(* Logix 5000 AddOnInstructionDefinition export Banner_Q90R2_KD_Param_v4; software revision 33.00; part 2 of 3 *)
(* tags used below, declared in another part *)
   Q90R2KD : Banner_Q90R2KD_v4;
   Port_Data : Banner_IOL_Port_v4;
   Port : DINT;
   Local_Control : DINT;
   Command_Being_Processed : BOOL;
   Inprocess_Index : DINT;
(* Banner_Q90R2_KD_Param_v4, continued *)

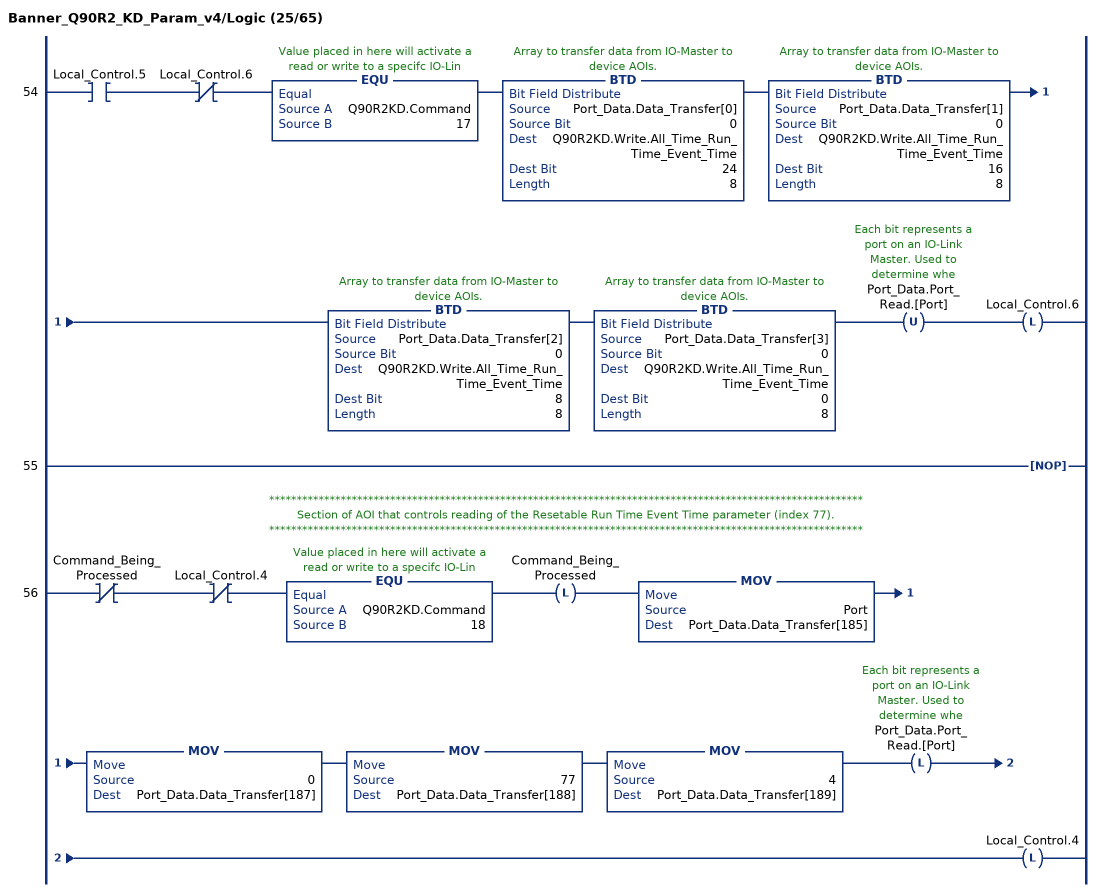
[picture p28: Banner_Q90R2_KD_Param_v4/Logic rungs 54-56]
   54: XIC(Local_Control.5)XIO(Local_Control.6)EQU(Q90R2KD.Command,17)BTD(Port_Data.Data_Transfer[0],0,Q90R2KD.Write.All_Time_Run_Time_Event_Time,24,8)BTD(Port_Data.Data_Transfer[1],0,Q90R2KD.Write.All_Time_Run_Time_Event_Time,16,8)BTD(Port_Data.Data_Transfer[2],0,Q90R2KD.Write.All_Time_Run_Time_Event_Time,8,8)BTD(Port_Data.Data_Transfer[3],0,Q90R2KD.Write.All_Time_Run_Time_Event_Time,0,8)OTU(Port_Data.Port_Read.[Port])OTL(Local_Control.6);
   55: NOP();
   // ************************************************************************************************************
   // Section of AOI that controls reading of the Resetable Run Time Event Time parameter (index 77).
   // ************************************************************************************************************
   56: XIO(Command_Being_Processed)XIO(Local_Control.4)EQU(Q90R2KD.Command,18)OTL(Command_Being_Processed)MOV(Port,Port_Data.Data_Transfer[185])MOV(0,Port_Data.Data_Transfer[187])MOV(77,Port_Data.Data_Transfer[188])MOV(4,Port_Data.Data_Transfer[189])OTL(Port_Data.Port_Read.[Port])OTL(Local_Control.4);
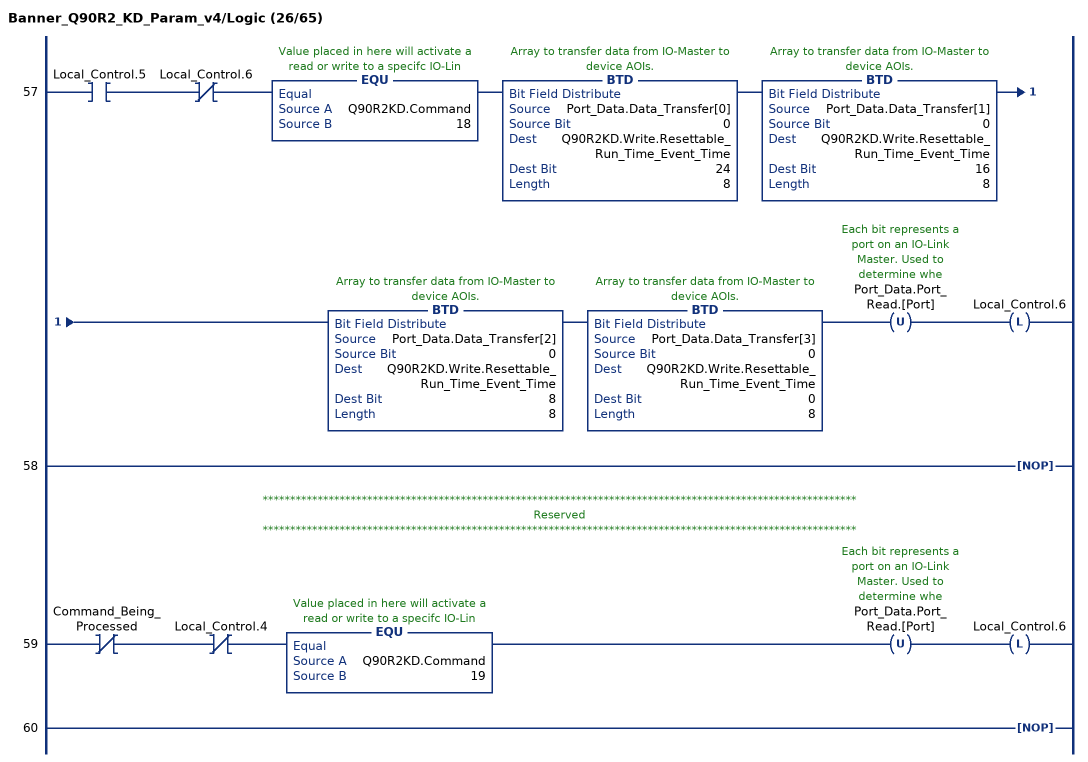
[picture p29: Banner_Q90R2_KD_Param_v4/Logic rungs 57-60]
   57: XIC(Local_Control.5)XIO(Local_Control.6)EQU(Q90R2KD.Command,18)BTD(Port_Data.Data_Transfer[0],0,Q90R2KD.Write.Resettable_Run_Time_Event_Time,24,8)BTD(Port_Data.Data_Transfer[1],0,Q90R2KD.Write.Resettable_Run_Time_Event_Time,16,8)BTD(Port_Data.Data_Transfer[2],0,Q90R2KD.Write.Resettable_Run_Time_Event_Time,8,8)BTD(Port_Data.Data_Transfer[3],0,Q90R2KD.Write.Resettable_Run_Time_Event_Time,0,8)OTU(Port_Data.Port_Read.[Port])OTL(Local_Control.6);
   58: NOP();
   // ************************************************************************************************************
   // Reserved
   // ************************************************************************************************************
   59: XIO(Command_Being_Processed)XIO(Local_Control.4)EQU(Q90R2KD.Command,19)OTU(Port_Data.Port_Read.[Port])OTL(Local_Control.6);
   60: NOP();
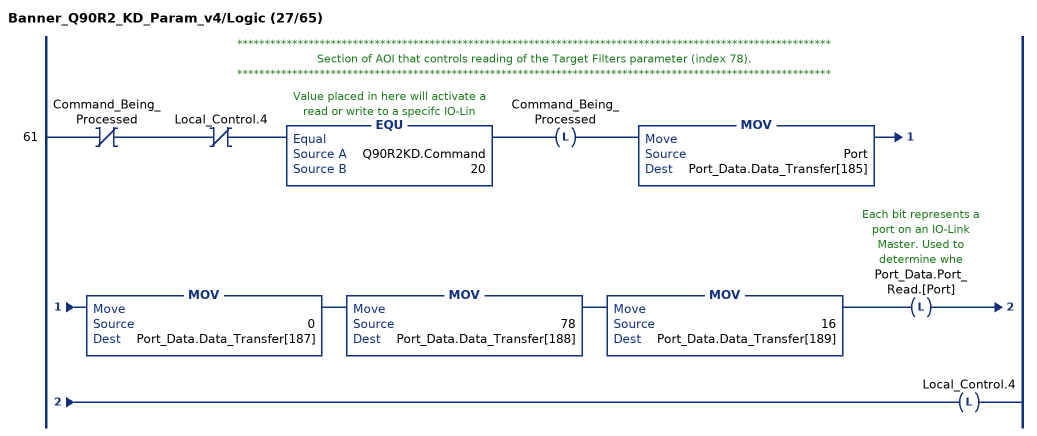
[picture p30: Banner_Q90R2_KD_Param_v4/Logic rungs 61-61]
   // ************************************************************************************************************
   // Section of AOI that controls reading of the Target Filters parameter (index 78).
   // ************************************************************************************************************
   61: XIO(Command_Being_Processed)XIO(Local_Control.4)EQU(Q90R2KD.Command,20)OTL(Command_Being_Processed)MOV(Port,Port_Data.Data_Transfer[185])MOV(0,Port_Data.Data_Transfer[187])MOV(78,Port_Data.Data_Transfer[188])MOV(16,Port_Data.Data_Transfer[189])OTL(Port_Data.Port_Read.[Port])OTL(Local_Control.4);
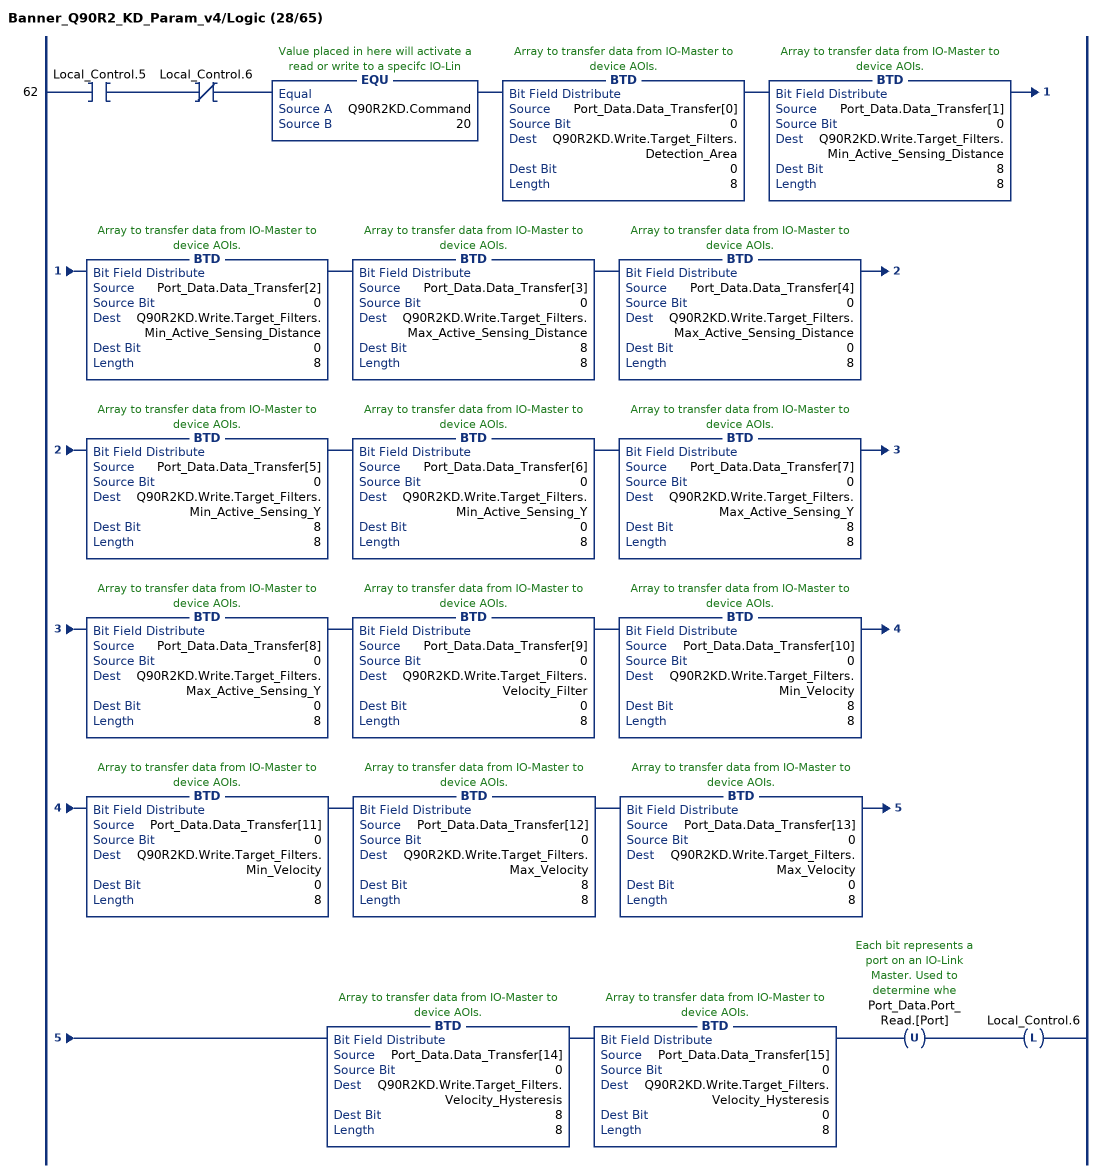
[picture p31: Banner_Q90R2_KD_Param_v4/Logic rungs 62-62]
   62: XIC(Local_Control.5)XIO(Local_Control.6)EQU(Q90R2KD.Command,20)BTD(Port_Data.Data_Transfer[0],0,Q90R2KD.Write.Target_Filters.Detection_Area,0,8)BTD(Port_Data.Data_Transfer[1],0,Q90R2KD.Write.Target_Filters.Min_Active_Sensing_Distance,8,8)BTD(Port_Data.Data_Transfer[2],0,Q90R2KD.Write.Target_Filters.Min_Active_Sensing_Distance,0,8)BTD(Port_Data.Data_Transfer[3],0,Q90R2KD.Write.Target_Filters.Max_Active_Sensing_Distance,8,8)BTD(Port_Data.Data_Transfer[4],0,Q90R2KD.Write.Target_Filters.Max_Active_Sensing_Distance,0,8)BTD(Port_Data.Data_Transfer[5],0,Q90R2KD.Write.Target_Filters.Min_Active_Sensing_Y,8,8)BTD(Port_Data.Data_Transfer[6],0,Q90R2KD.Write.Target_Filters.Min_Active_Sensing_Y,0,8)BTD(Port_Data.Data_Transfer[7],0,Q90R2KD.Write.Target_Filters.Max_Active_Sensing_Y,8,8)BTD(Port_Data.Data_Transfer[8],0,Q90R2KD.Write.Target_Filters.Max_Active_Sensing_Y,0,8)BTD(Port_Data.Data_Transfer[9],0,Q90R2KD.Write.Target_Filters.Velocity_Filter,0,8)BTD(Port_Data.Data_Transfer[10],0,Q90R2KD.Write.Target_Filters.Min_Velocity,8,8)BTD(Port_Data.Data_Transfer[11],0,Q90R2KD.Write.Target_Filters.Min_Velocity,0,8)BTD(Port_Data.Data_Transfer[12],0,Q90R2KD.Write.Target_Filters.Max_Velocity,8,8)BTD(Port_Data.Data_Transfer[13],0,Q90R2KD.Write.Target_Filters.Max_Velocity,0,8)BTD(Port_Data.Data_Transfer[14],0,Q90R2KD.Write.Target_Filters.Velocity_Hysteresis,8,8)BTD(Port_Data.Data_Transfer[15],0,Q90R2KD.Write.Target_Filters.Velocity_Hysteresis,0,8)OTU(Port_Data.Port_Read.[Port])OTL(Local_Control.6);
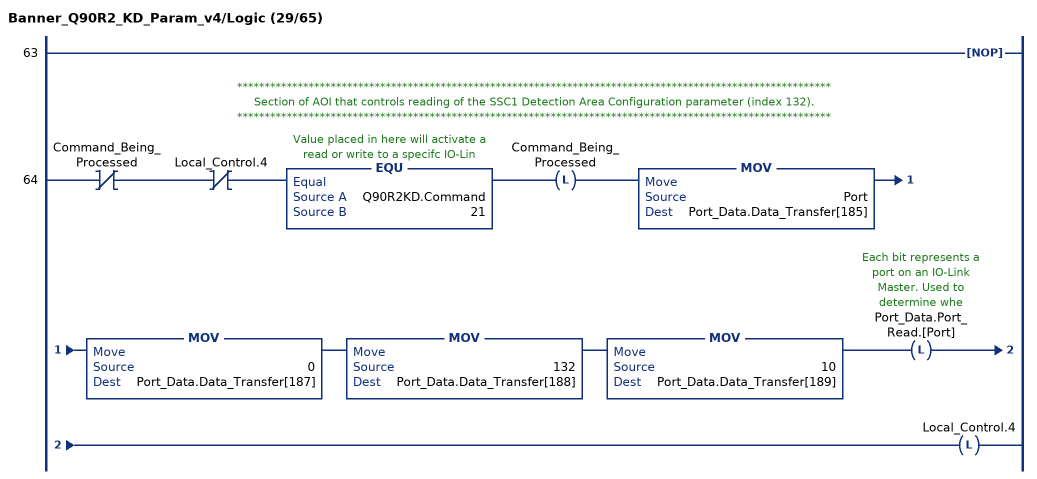
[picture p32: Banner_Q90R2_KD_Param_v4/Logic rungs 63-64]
   63: NOP();
   // ************************************************************************************************************
   // Section of AOI that controls reading of the SSC1 Detection Area Configuration parameter (index 132).
   // ************************************************************************************************************
   64: XIO(Command_Being_Processed)XIO(Local_Control.4)EQU(Q90R2KD.Command,21)OTL(Command_Being_Processed)MOV(Port,Port_Data.Data_Transfer[185])MOV(0,Port_Data.Data_Transfer[187])MOV(132,Port_Data.Data_Transfer[188])MOV(10,Port_Data.Data_Transfer[189])OTL(Port_Data.Port_Read.[Port])OTL(Local_Control.4);
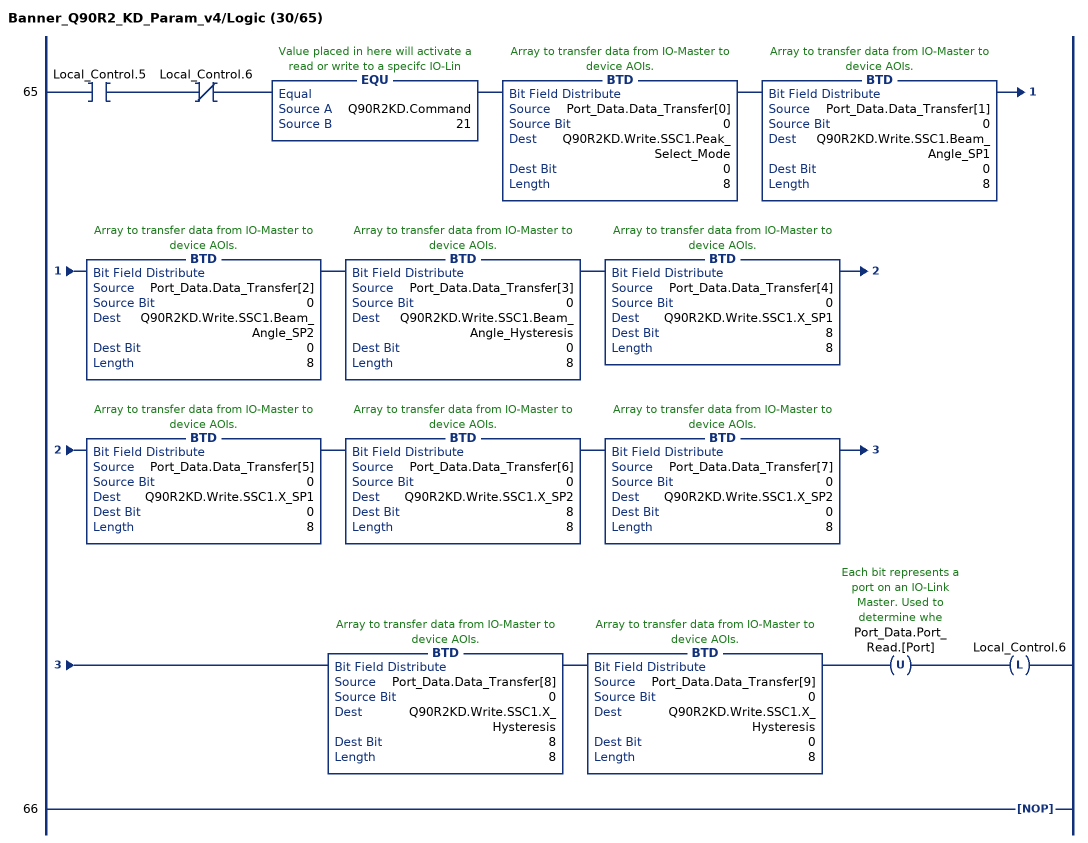
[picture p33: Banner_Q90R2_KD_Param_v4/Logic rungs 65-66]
   65: XIC(Local_Control.5)XIO(Local_Control.6)EQU(Q90R2KD.Command,21)BTD(Port_Data.Data_Transfer[0],0,Q90R2KD.Write.SSC1.Peak_Select_Mode,0,8)BTD(Port_Data.Data_Transfer[1],0,Q90R2KD.Write.SSC1.Beam_Angle_SP1,0,8)BTD(Port_Data.Data_Transfer[2],0,Q90R2KD.Write.SSC1.Beam_Angle_SP2,0,8)BTD(Port_Data.Data_Transfer[3],0,Q90R2KD.Write.SSC1.Beam_Angle_Hysteresis,0,8)BTD(Port_Data.Data_Transfer[4],0,Q90R2KD.Write.SSC1.X_SP1,8,8)BTD(Port_Data.Data_Transfer[5],0,Q90R2KD.Write.SSC1.X_SP1,0,8)BTD(Port_Data.Data_Transfer[6],0,Q90R2KD.Write.SSC1.X_SP2,8,8)BTD(Port_Data.Data_Transfer[7],0,Q90R2KD.Write.SSC1.X_SP2,0,8)BTD(Port_Data.Data_Transfer[8],0,Q90R2KD.Write.SSC1.X_Hysteresis,8,8)BTD(Port_Data.Data_Transfer[9],0,Q90R2KD.Write.SSC1.X_Hysteresis,0,8)OTU(Port_Data.Port_Read.[Port])OTL(Local_Control.6);
   66: NOP();
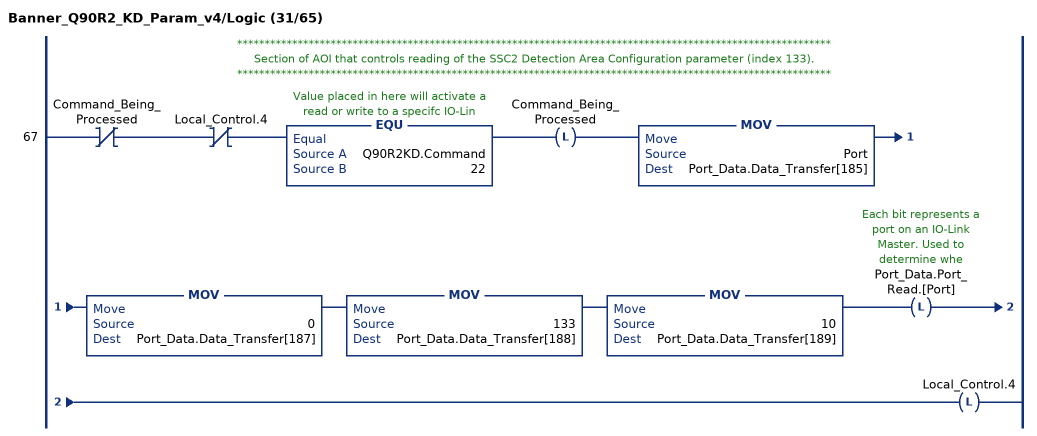
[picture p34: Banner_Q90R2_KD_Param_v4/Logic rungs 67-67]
   // ************************************************************************************************************
   // Section of AOI that controls reading of the SSC2 Detection Area Configuration parameter (index 133).
   // ************************************************************************************************************
   67: XIO(Command_Being_Processed)XIO(Local_Control.4)EQU(Q90R2KD.Command,22)OTL(Command_Being_Processed)MOV(Port,Port_Data.Data_Transfer[185])MOV(0,Port_Data.Data_Transfer[187])MOV(133,Port_Data.Data_Transfer[188])MOV(10,Port_Data.Data_Transfer[189])OTL(Port_Data.Port_Read.[Port])OTL(Local_Control.4);
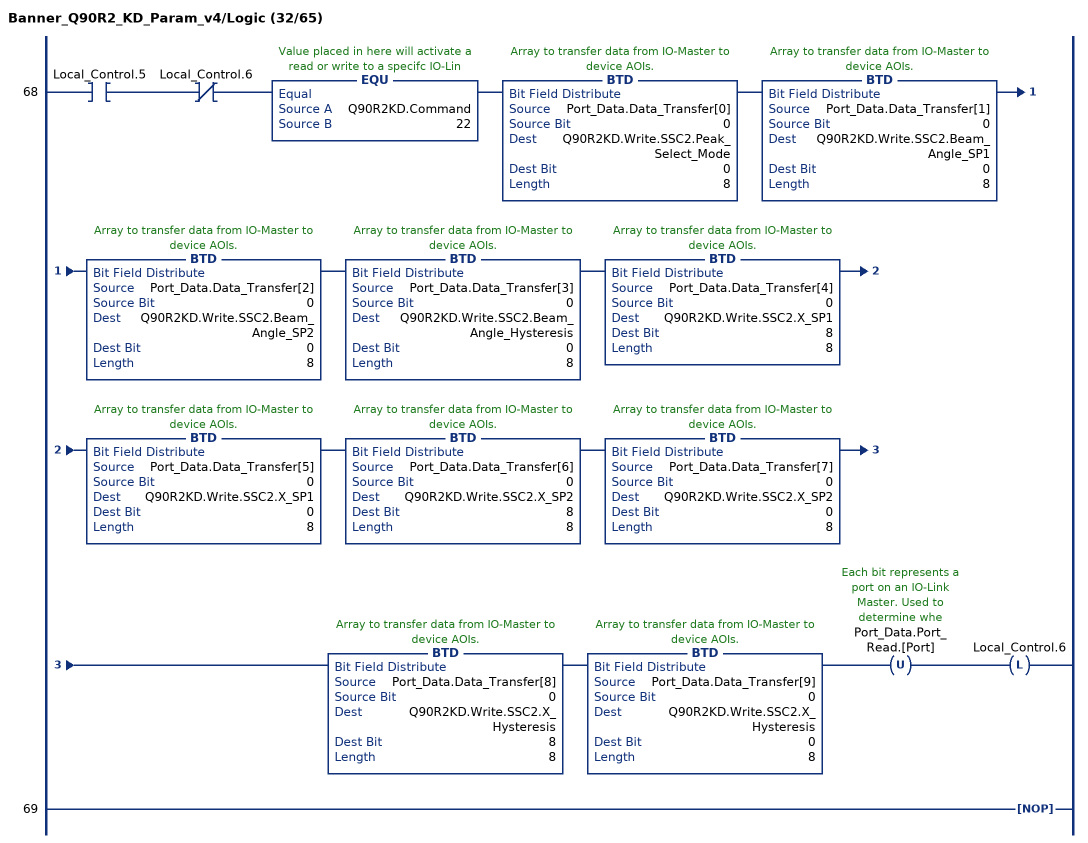
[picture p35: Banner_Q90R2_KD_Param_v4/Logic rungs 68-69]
   68: XIC(Local_Control.5)XIO(Local_Control.6)EQU(Q90R2KD.Command,22)BTD(Port_Data.Data_Transfer[0],0,Q90R2KD.Write.SSC2.Peak_Select_Mode,0,8)BTD(Port_Data.Data_Transfer[1],0,Q90R2KD.Write.SSC2.Beam_Angle_SP1,0,8)BTD(Port_Data.Data_Transfer[2],0,Q90R2KD.Write.SSC2.Beam_Angle_SP2,0,8)BTD(Port_Data.Data_Transfer[3],0,Q90R2KD.Write.SSC2.Beam_Angle_Hysteresis,0,8)BTD(Port_Data.Data_Transfer[4],0,Q90R2KD.Write.SSC2.X_SP1,8,8)BTD(Port_Data.Data_Transfer[5],0,Q90R2KD.Write.SSC2.X_SP1,0,8)BTD(Port_Data.Data_Transfer[6],0,Q90R2KD.Write.SSC2.X_SP2,8,8)BTD(Port_Data.Data_Transfer[7],0,Q90R2KD.Write.SSC2.X_SP2,0,8)BTD(Port_Data.Data_Transfer[8],0,Q90R2KD.Write.SSC2.X_Hysteresis,8,8)BTD(Port_Data.Data_Transfer[9],0,Q90R2KD.Write.SSC2.X_Hysteresis,0,8)OTU(Port_Data.Port_Read.[Port])OTL(Local_Control.6);
   69: NOP();
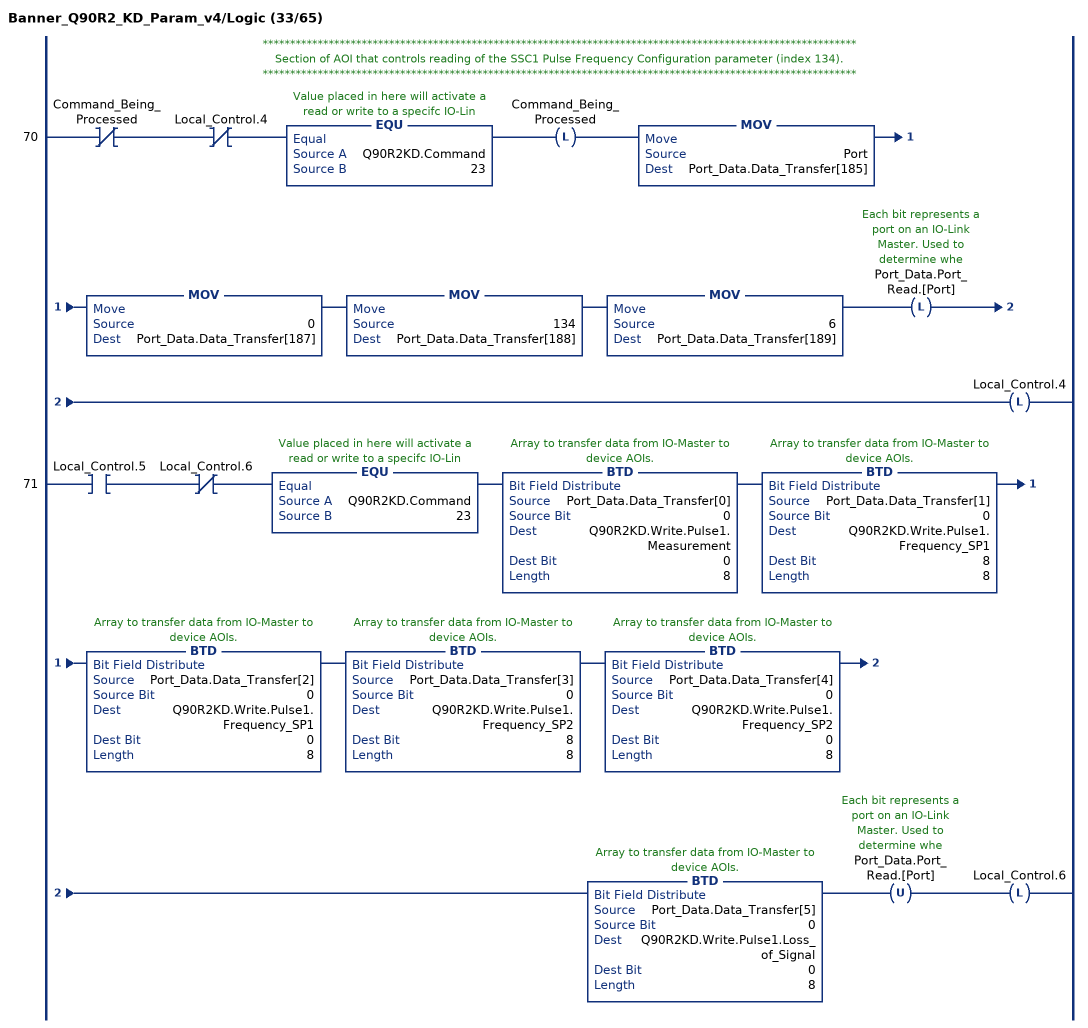
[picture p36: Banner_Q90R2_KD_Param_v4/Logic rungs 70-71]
   // ************************************************************************************************************
   // Section of AOI that controls reading of the SSC1 Pulse Frequency Configuration parameter (index 134).
   // ************************************************************************************************************
   70: XIO(Command_Being_Processed)XIO(Local_Control.4)EQU(Q90R2KD.Command,23)OTL(Command_Being_Processed)MOV(Port,Port_Data.Data_Transfer[185])MOV(0,Port_Data.Data_Transfer[187])MOV(134,Port_Data.Data_Transfer[188])MOV(6,Port_Data.Data_Transfer[189])OTL(Port_Data.Port_Read.[Port])OTL(Local_Control.4);
   71: XIC(Local_Control.5)XIO(Local_Control.6)EQU(Q90R2KD.Command,23)BTD(Port_Data.Data_Transfer[0],0,Q90R2KD.Write.Pulse1.Measurement,0,8)BTD(Port_Data.Data_Transfer[1],0,Q90R2KD.Write.Pulse1.Frequency_SP1,8,8)BTD(Port_Data.Data_Transfer[2],0,Q90R2KD.Write.Pulse1.Frequency_SP1,0,8)BTD(Port_Data.Data_Transfer[3],0,Q90R2KD.Write.Pulse1.Frequency_SP2,8,8)BTD(Port_Data.Data_Transfer[4],0,Q90R2KD.Write.Pulse1.Frequency_SP2,0,8)BTD(Port_Data.Data_Transfer[5],0,Q90R2KD.Write.Pulse1.Loss_of_Signal,0,8)OTU(Port_Data.Port_Read.[Port])OTL(Local_Control.6);
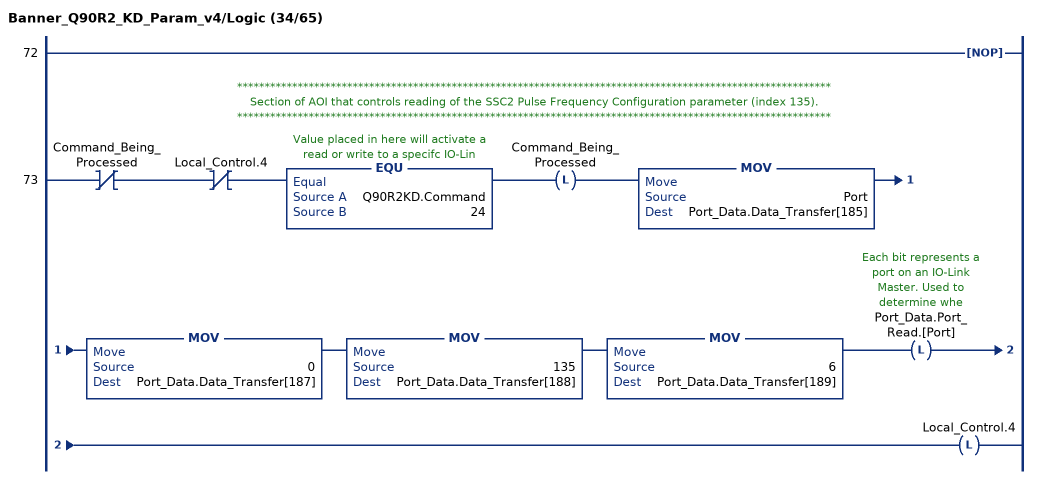
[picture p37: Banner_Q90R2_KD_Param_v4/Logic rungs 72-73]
   72: NOP();
   // ************************************************************************************************************
   // Section of AOI that controls reading of the SSC2 Pulse Frequency Configuration parameter (index 135).
   // ************************************************************************************************************
   73: XIO(Command_Being_Processed)XIO(Local_Control.4)EQU(Q90R2KD.Command,24)OTL(Command_Being_Processed)MOV(Port,Port_Data.Data_Transfer[185])MOV(0,Port_Data.Data_Transfer[187])MOV(135,Port_Data.Data_Transfer[188])MOV(6,Port_Data.Data_Transfer[189])OTL(Port_Data.Port_Read.[Port])OTL(Local_Control.4);
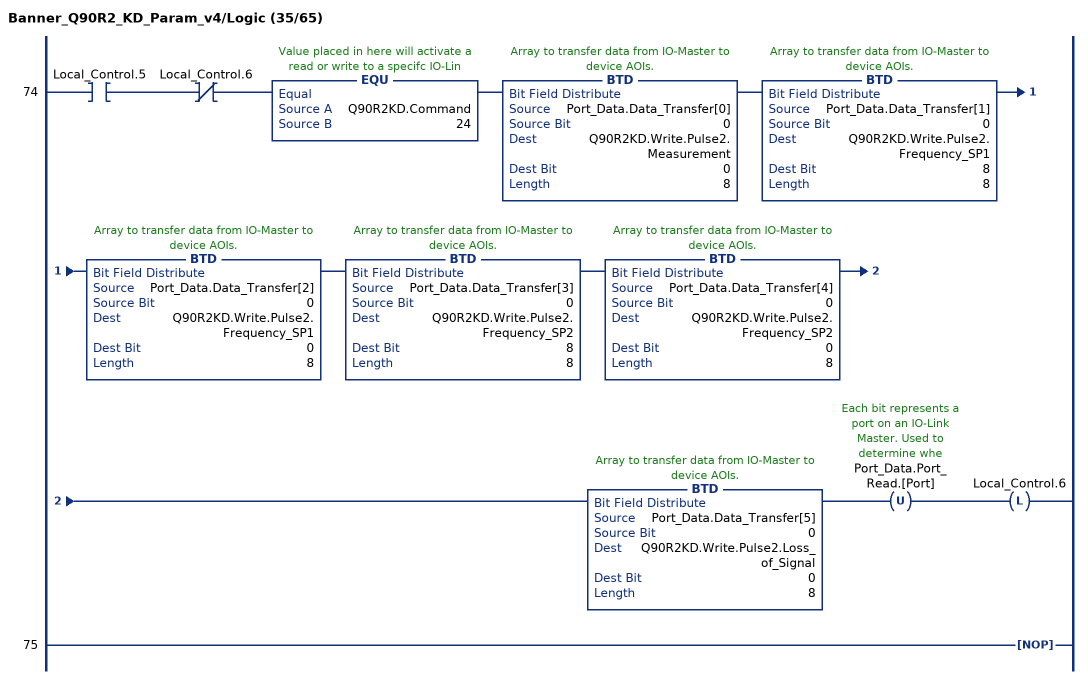
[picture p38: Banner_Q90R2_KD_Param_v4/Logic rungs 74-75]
   74: XIC(Local_Control.5)XIO(Local_Control.6)EQU(Q90R2KD.Command,24)BTD(Port_Data.Data_Transfer[0],0,Q90R2KD.Write.Pulse2.Measurement,0,8)BTD(Port_Data.Data_Transfer[1],0,Q90R2KD.Write.Pulse2.Frequency_SP1,8,8)BTD(Port_Data.Data_Transfer[2],0,Q90R2KD.Write.Pulse2.Frequency_SP1,0,8)BTD(Port_Data.Data_Transfer[3],0,Q90R2KD.Write.Pulse2.Frequency_SP2,8,8)BTD(Port_Data.Data_Transfer[4],0,Q90R2KD.Write.Pulse2.Frequency_SP2,0,8)BTD(Port_Data.Data_Transfer[5],0,Q90R2KD.Write.Pulse2.Loss_of_Signal,0,8)OTU(Port_Data.Port_Read.[Port])OTL(Local_Control.6);
   75: NOP();
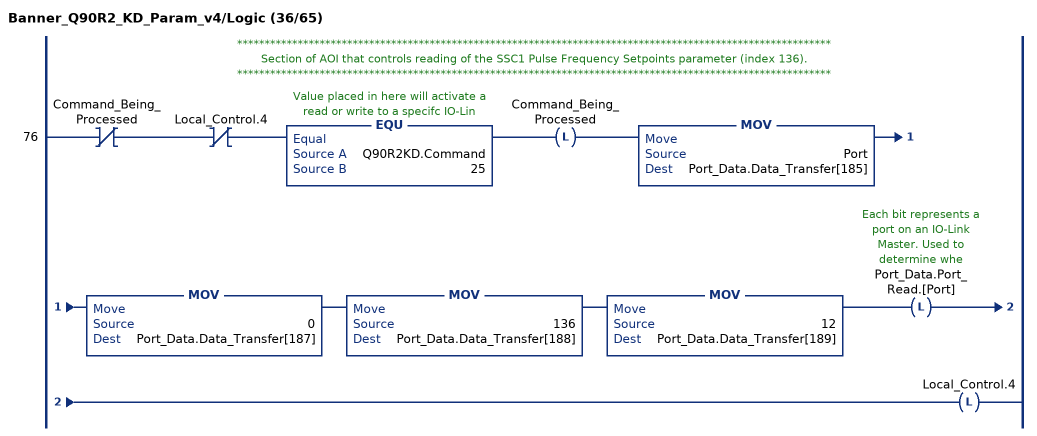
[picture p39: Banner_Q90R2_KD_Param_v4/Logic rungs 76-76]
   // ************************************************************************************************************
   // Section of AOI that controls reading of the SSC1 Pulse Frequency Setpoints parameter (index 136).
   // ************************************************************************************************************
   76: XIO(Command_Being_Processed)XIO(Local_Control.4)EQU(Q90R2KD.Command,25)OTL(Command_Being_Processed)MOV(Port,Port_Data.Data_Transfer[185])MOV(0,Port_Data.Data_Transfer[187])MOV(136,Port_Data.Data_Transfer[188])MOV(12,Port_Data.Data_Transfer[189])OTL(Port_Data.Port_Read.[Port])OTL(Local_Control.4);
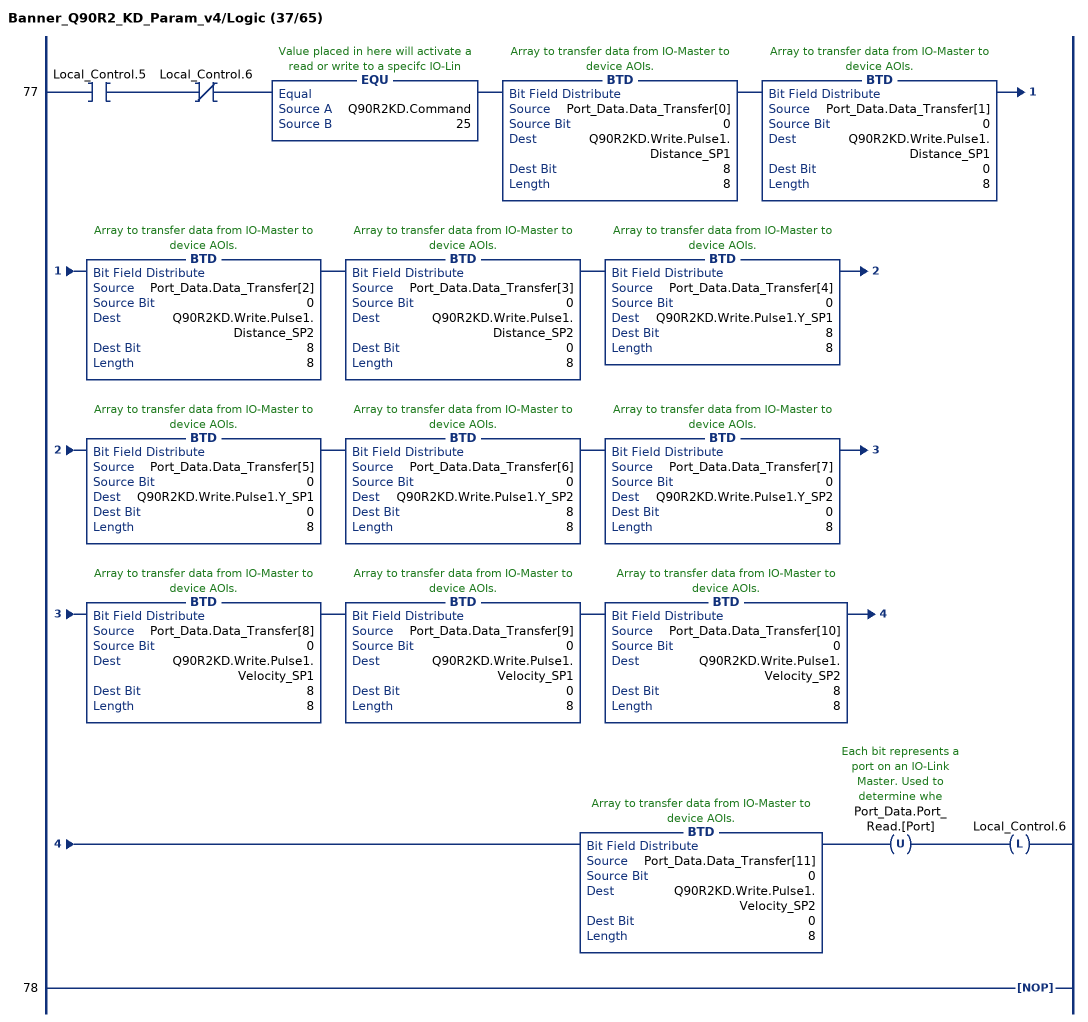
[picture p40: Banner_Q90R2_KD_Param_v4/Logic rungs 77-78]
   77: XIC(Local_Control.5)XIO(Local_Control.6)EQU(Q90R2KD.Command,25)BTD(Port_Data.Data_Transfer[0],0,Q90R2KD.Write.Pulse1.Distance_SP1,8,8)BTD(Port_Data.Data_Transfer[1],0,Q90R2KD.Write.Pulse1.Distance_SP1,0,8)BTD(Port_Data.Data_Transfer[2],0,Q90R2KD.Write.Pulse1.Distance_SP2,8,8)BTD(Port_Data.Data_Transfer[3],0,Q90R2KD.Write.Pulse1.Distance_SP2,0,8)BTD(Port_Data.Data_Transfer[4],0,Q90R2KD.Write.Pulse1.Y_SP1,8,8)BTD(Port_Data.Data_Transfer[5],0,Q90R2KD.Write.Pulse1.Y_SP1,0,8)BTD(Port_Data.Data_Transfer[6],0,Q90R2KD.Write.Pulse1.Y_SP2,8,8)BTD(Port_Data.Data_Transfer[7],0,Q90R2KD.Write.Pulse1.Y_SP2,0,8)BTD(Port_Data.Data_Transfer[8],0,Q90R2KD.Write.Pulse1.Velocity_SP1,8,8)BTD(Port_Data.Data_Transfer[9],0,Q90R2KD.Write.Pulse1.Velocity_SP1,0,8)BTD(Port_Data.Data_Transfer[10],0,Q90R2KD.Write.Pulse1.Velocity_SP2,8,8)BTD(Port_Data.Data_Transfer[11],0,Q90R2KD.Write.Pulse1.Velocity_SP2,0,8)OTU(Port_Data.Port_Read.[Port])OTL(Local_Control.6);
   78: NOP();
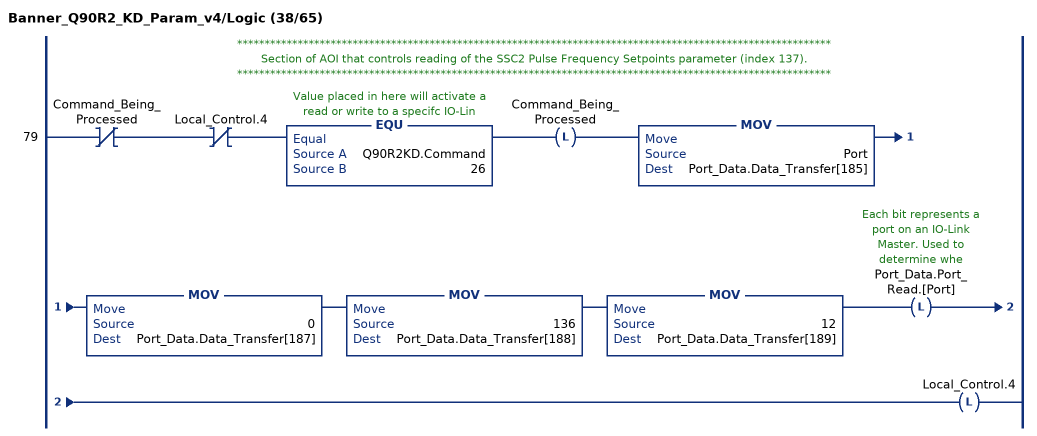
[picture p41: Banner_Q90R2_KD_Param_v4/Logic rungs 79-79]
   // ************************************************************************************************************
   // Section of AOI that controls reading of the SSC2 Pulse Frequency Setpoints parameter (index 137).
   // ************************************************************************************************************
   79: XIO(Command_Being_Processed)XIO(Local_Control.4)EQU(Q90R2KD.Command,26)OTL(Command_Being_Processed)MOV(Port,Port_Data.Data_Transfer[185])MOV(0,Port_Data.Data_Transfer[187])MOV(136,Port_Data.Data_Transfer[188])MOV(12,Port_Data.Data_Transfer[189])OTL(Port_Data.Port_Read.[Port])OTL(Local_Control.4);
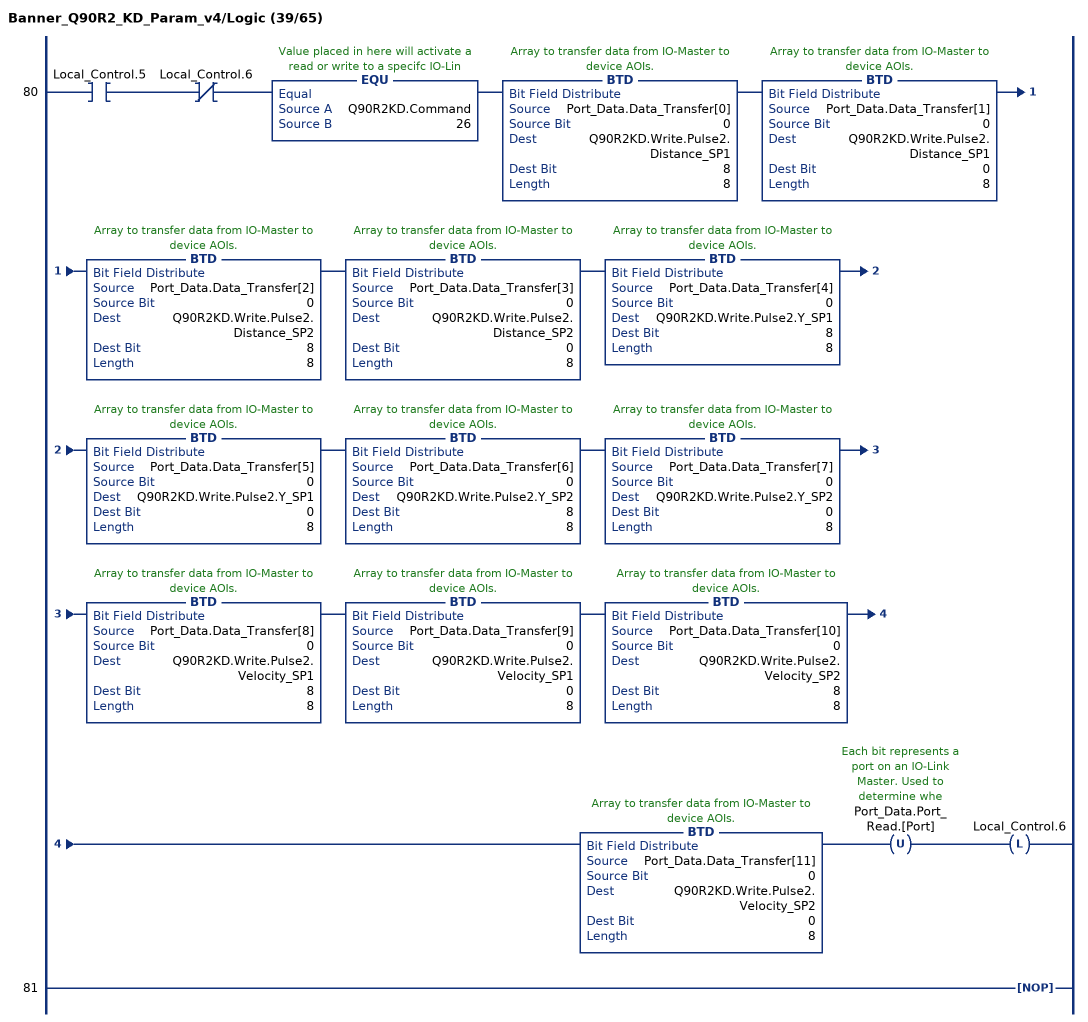
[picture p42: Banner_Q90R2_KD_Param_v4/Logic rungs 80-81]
   80: XIC(Local_Control.5)XIO(Local_Control.6)EQU(Q90R2KD.Command,26)BTD(Port_Data.Data_Transfer[0],0,Q90R2KD.Write.Pulse2.Distance_SP1,8,8)BTD(Port_Data.Data_Transfer[1],0,Q90R2KD.Write.Pulse2.Distance_SP1,0,8)BTD(Port_Data.Data_Transfer[2],0,Q90R2KD.Write.Pulse2.Distance_SP2,8,8)BTD(Port_Data.Data_Transfer[3],0,Q90R2KD.Write.Pulse2.Distance_SP2,0,8)BTD(Port_Data.Data_Transfer[4],0,Q90R2KD.Write.Pulse2.Y_SP1,8,8)BTD(Port_Data.Data_Transfer[5],0,Q90R2KD.Write.Pulse2.Y_SP1,0,8)BTD(Port_Data.Data_Transfer[6],0,Q90R2KD.Write.Pulse2.Y_SP2,8,8)BTD(Port_Data.Data_Transfer[7],0,Q90R2KD.Write.Pulse2.Y_SP2,0,8)BTD(Port_Data.Data_Transfer[8],0,Q90R2KD.Write.Pulse2.Velocity_SP1,8,8)BTD(Port_Data.Data_Transfer[9],0,Q90R2KD.Write.Pulse2.Velocity_SP1,0,8)BTD(Port_Data.Data_Transfer[10],0,Q90R2KD.Write.Pulse2.Velocity_SP2,8,8)BTD(Port_Data.Data_Transfer[11],0,Q90R2KD.Write.Pulse2.Velocity_SP2,0,8)OTU(Port_Data.Port_Read.[Port])OTL(Local_Control.6);
   81: NOP();
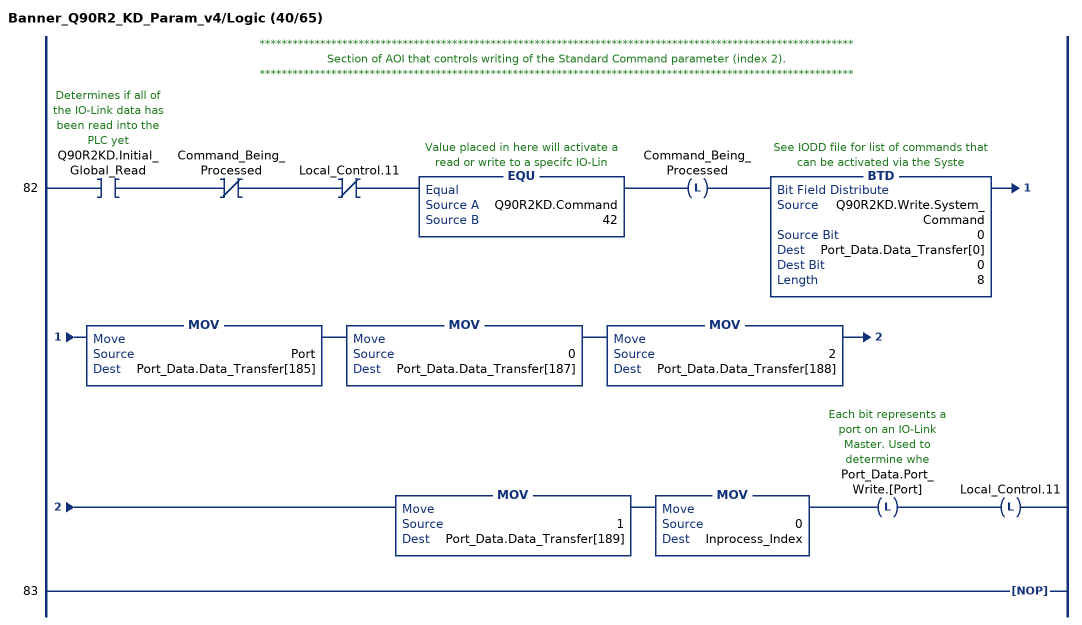
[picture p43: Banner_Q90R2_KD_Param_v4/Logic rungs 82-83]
   // ************************************************************************************************************
   // Section of AOI that controls writing of the Standard Command parameter (index 2).
   // ************************************************************************************************************
   82: XIC(Q90R2KD.Initial_Global_Read)XIO(Command_Being_Processed)XIO(Local_Control.11)EQU(Q90R2KD.Command,42)OTL(Command_Being_Processed)BTD(Q90R2KD.Write.System_Command,0,Port_Data.Data_Transfer[0],0,8)MOV(Port,Port_Data.Data_Transfer[185])MOV(0,Port_Data.Data_Transfer[187])MOV(2,Port_Data.Data_Transfer[188])MOV(1,Port_Data.Data_Transfer[189])MOV(0,Inprocess_Index)OTL(Port_Data.Port_Write.[Port])OTL(Local_Control.11);
   83: NOP();
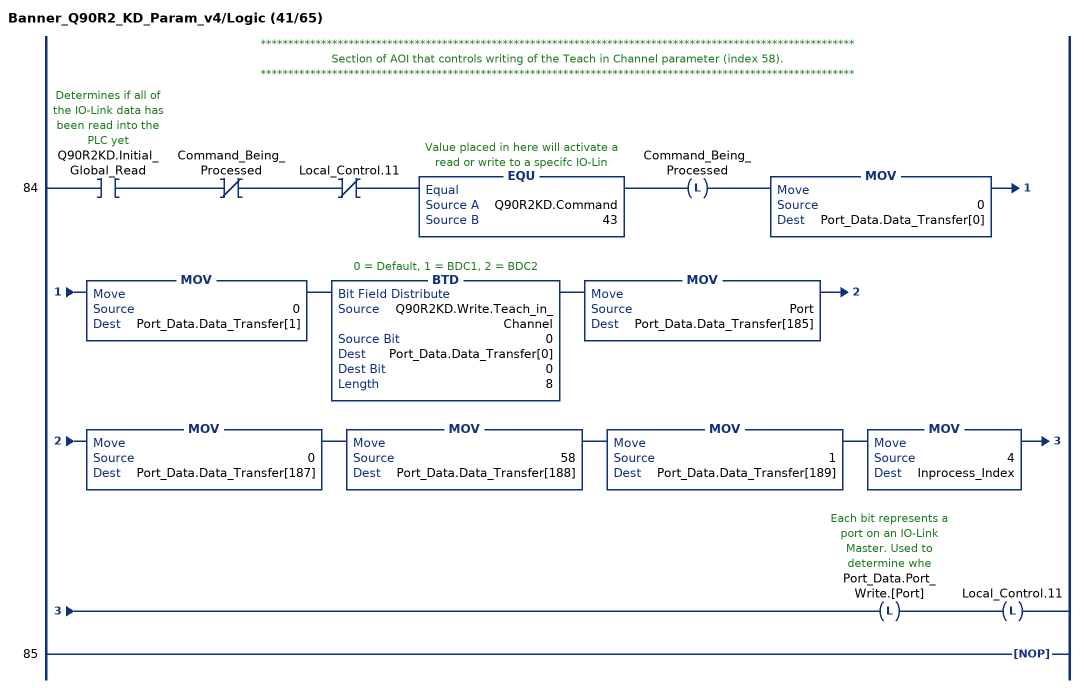
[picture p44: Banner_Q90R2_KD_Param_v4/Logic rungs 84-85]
   // ************************************************************************************************************
   // Section of AOI that controls writing of the Teach in Channel parameter (index 58).
   // ************************************************************************************************************
   84: XIC(Q90R2KD.Initial_Global_Read)XIO(Command_Being_Processed)XIO(Local_Control.11)EQU(Q90R2KD.Command,43)OTL(Command_Being_Processed)MOV(0,Port_Data.Data_Transfer[0])MOV(0,Port_Data.Data_Transfer[1])BTD(Q90R2KD.Write.Teach_in_Channel,0,Port_Data.Data_Transfer[0],0,8)MOV(Port,Port_Data.Data_Transfer[185])MOV(0,Port_Data.Data_Transfer[187])MOV(58,Port_Data.Data_Transfer[188])MOV(1,Port_Data.Data_Transfer[189])MOV(4,Inprocess_Index)OTL(Port_Data.Port_Write.[Port])OTL(Local_Control.11);
   85: NOP();
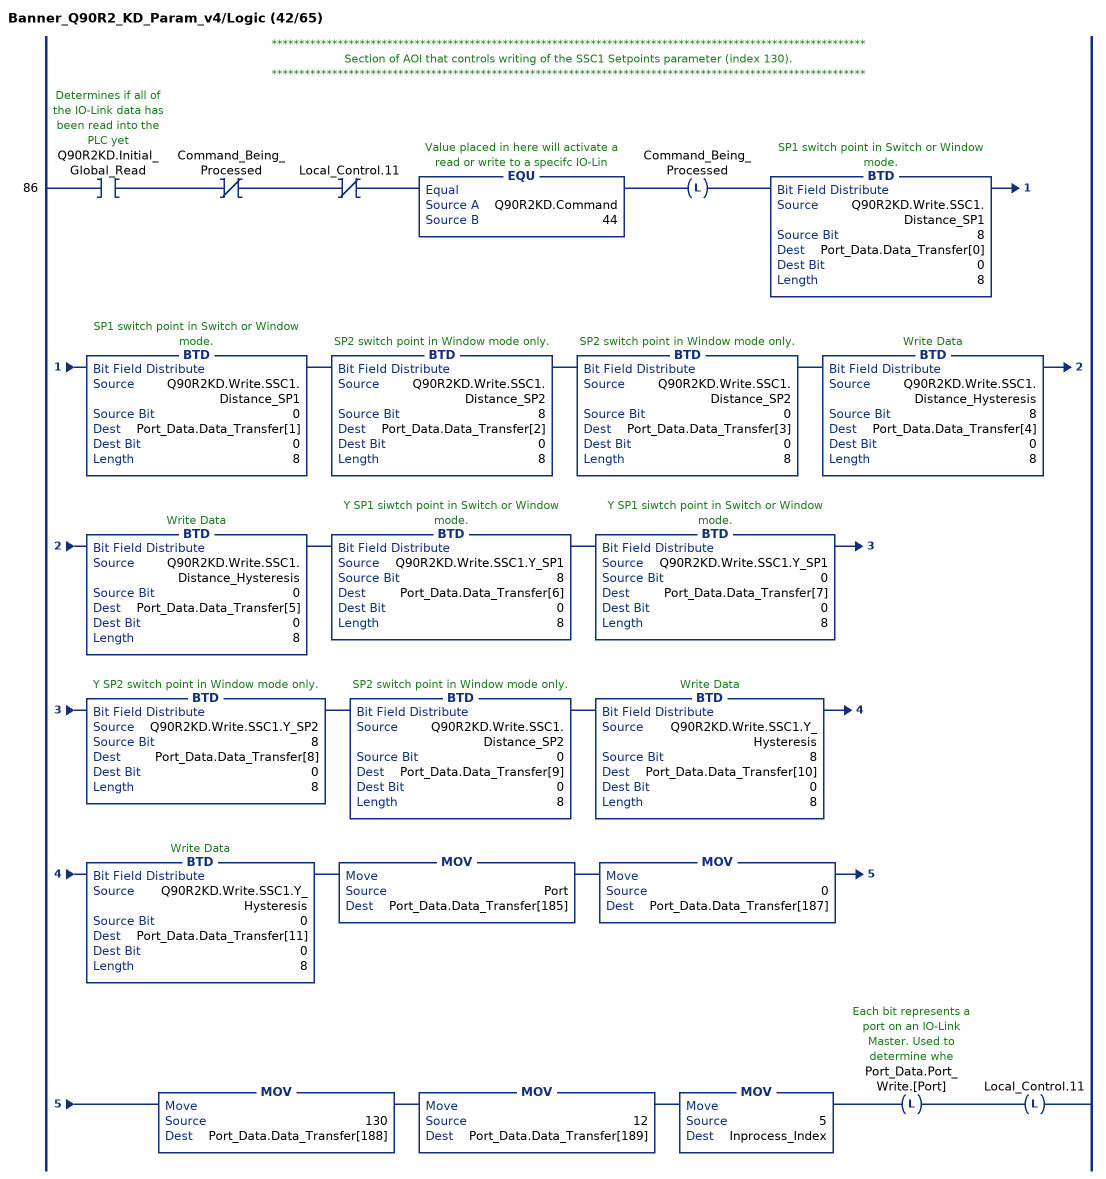
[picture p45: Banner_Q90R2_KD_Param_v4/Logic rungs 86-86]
   // ************************************************************************************************************
   // Section of AOI that controls writing of the SSC1 Setpoints parameter (index 130).
   // ************************************************************************************************************
   86: XIC(Q90R2KD.Initial_Global_Read)XIO(Command_Being_Processed)XIO(Local_Control.11)EQU(Q90R2KD.Command,44)OTL(Command_Being_Processed)BTD(Q90R2KD.Write.SSC1.Distance_SP1,8,Port_Data.Data_Transfer[0],0,8)BTD(Q90R2KD.Write.SSC1.Distance_SP1,0,Port_Data.Data_Transfer[1],0,8)BTD(Q90R2KD.Write.SSC1.Distance_SP2,8,Port_Data.Data_Transfer[2],0,8)BTD(Q90R2KD.Write.SSC1.Distance_SP2,0,Port_Data.Data_Transfer[3],0,8)BTD(Q90R2KD.Write.SSC1.Distance_Hysteresis,8,Port_Data.Data_Transfer[4],0,8)BTD(Q90R2KD.Write.SSC1.Distance_Hysteresis,0,Port_Data.Data_Transfer[5],0,8)BTD(Q90R2KD.Write.SSC1.Y_SP1,8,Port_Data.Data_Transfer[6],0,8)BTD(Q90R2KD.Write.SSC1.Y_SP1,0,Port_Data.Data_Transfer[7],0,8)BTD(Q90R2KD.Write.SSC1.Y_SP2,8,Port_Data.Data_Transfer[8],0,8)BTD(Q90R2KD.Write.SSC1.Distance_SP2,0,Port_Data.Data_Transfer[9],0,8)BTD(Q90R2KD.Write.SSC1.Y_Hysteresis,8,Port_Data.Data_Transfer[10],0,8)BTD(Q90R2KD.Write.SSC1.Y_Hysteresis,0,Port_Data.Data_Transfer[11],0,8)MOV(Port,Port_Data.Data_Transfer[185])MOV(0,Port_Data.Data_Transfer[187])MOV(130,Port_Data.Data_Transfer[188])MOV(12,Port_Data.Data_Transfer[189])MOV(5,Inprocess_Index)OTL(Port_Data.Port_Write.[Port])OTL(Local_Control.11);
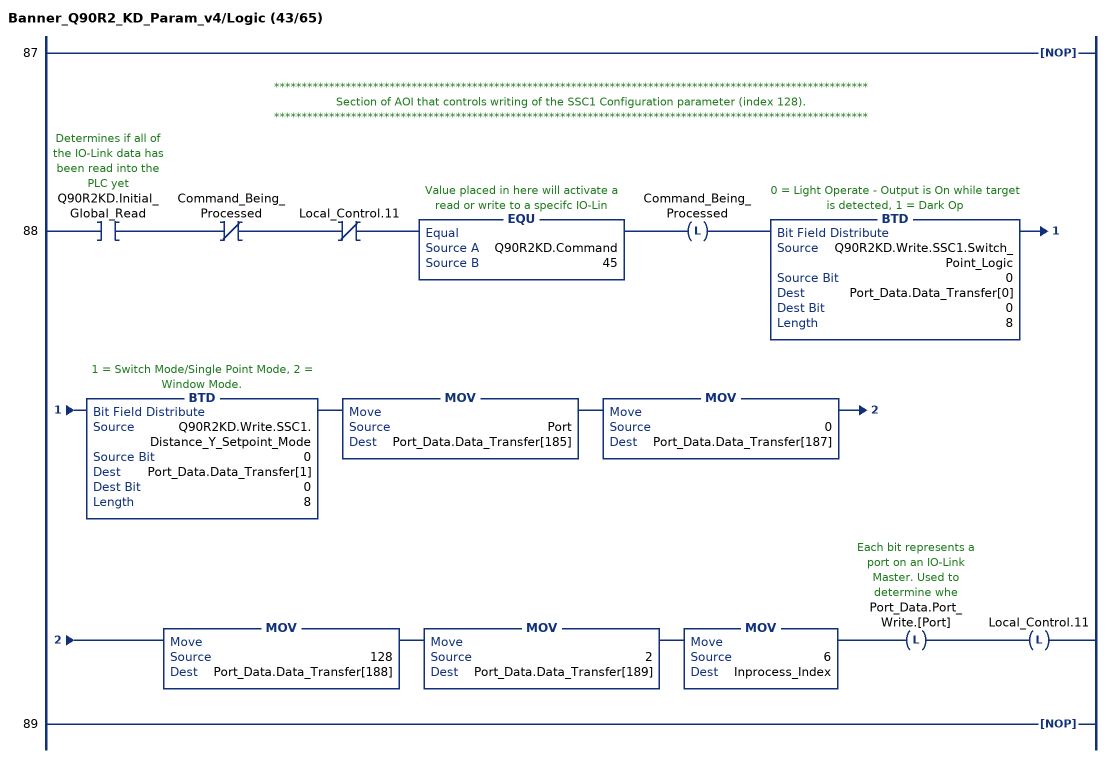
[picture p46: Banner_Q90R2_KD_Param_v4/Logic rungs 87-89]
   87: NOP();
   // ************************************************************************************************************
   // Section of AOI that controls writing of the SSC1 Configuration parameter (index 128).
   // ************************************************************************************************************
   88: XIC(Q90R2KD.Initial_Global_Read)XIO(Command_Being_Processed)XIO(Local_Control.11)EQU(Q90R2KD.Command,45)OTL(Command_Being_Processed)BTD(Q90R2KD.Write.SSC1.Switch_Point_Logic,0,Port_Data.Data_Transfer[0],0,8)BTD(Q90R2KD.Write.SSC1.Distance_Y_Setpoint_Mode,0,Port_Data.Data_Transfer[1],0,8)MOV(Port,Port_Data.Data_Transfer[185])MOV(0,Port_Data.Data_Transfer[187])MOV(128,Port_Data.Data_Transfer[188])MOV(2,Port_Data.Data_Transfer[189])MOV(6,Inprocess_Index)OTL(Port_Data.Port_Write.[Port])OTL(Local_Control.11);
   89: NOP();
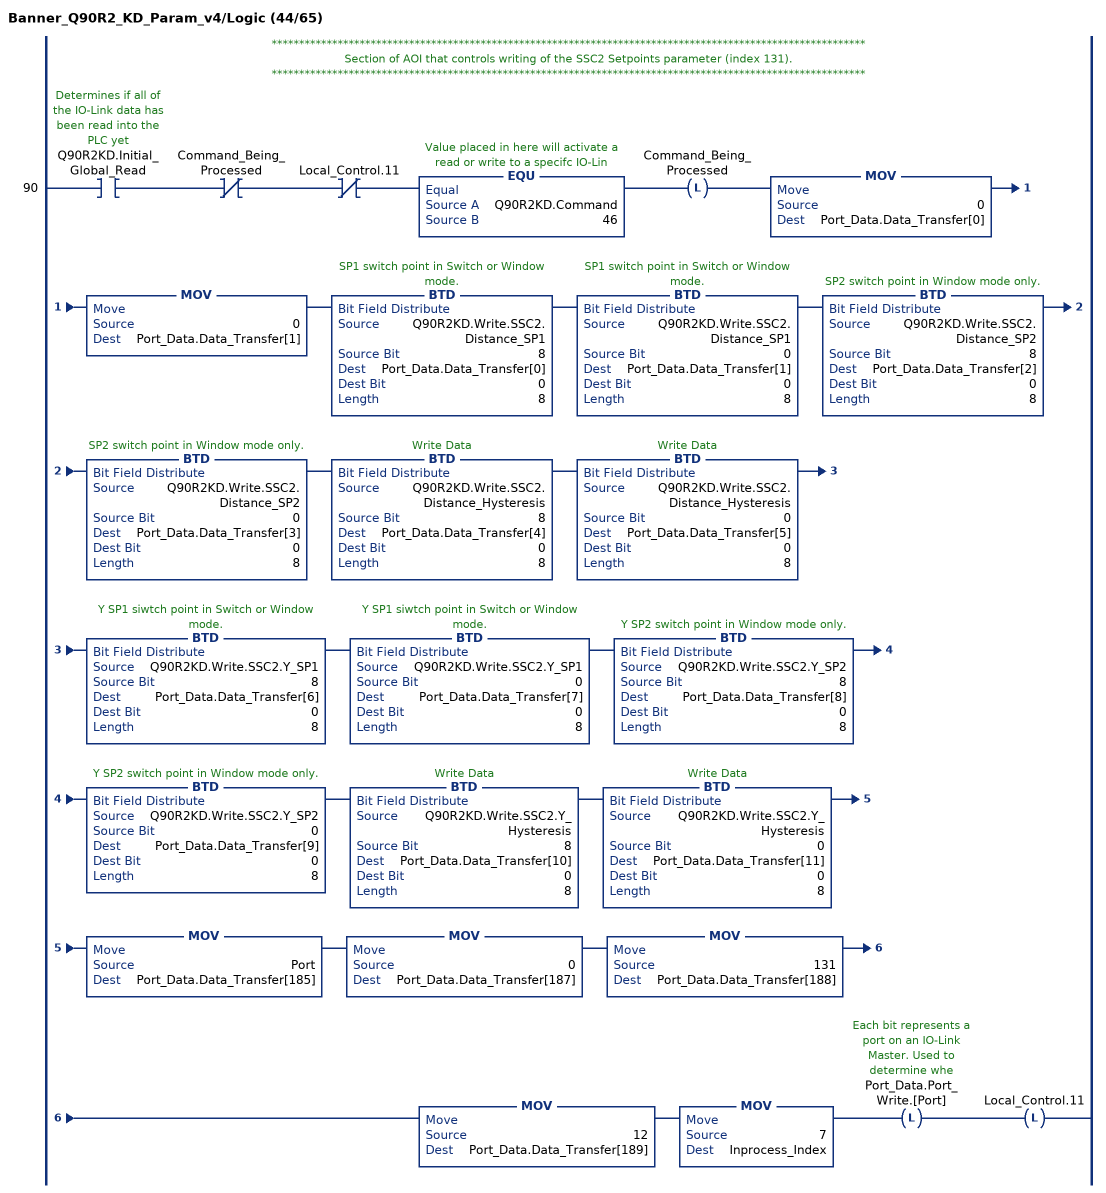
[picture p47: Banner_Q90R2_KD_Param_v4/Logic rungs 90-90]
   // ************************************************************************************************************
   // Section of AOI that controls writing of the SSC2 Setpoints parameter (index 131).
   // ************************************************************************************************************
   90: XIC(Q90R2KD.Initial_Global_Read)XIO(Command_Being_Processed)XIO(Local_Control.11)EQU(Q90R2KD.Command,46)OTL(Command_Being_Processed)MOV(0,Port_Data.Data_Transfer[0])MOV(0,Port_Data.Data_Transfer[1])BTD(Q90R2KD.Write.SSC2.Distance_SP1,8,Port_Data.Data_Transfer[0],0,8)BTD(Q90R2KD.Write.SSC2.Distance_SP1,0,Port_Data.Data_Transfer[1],0,8)BTD(Q90R2KD.Write.SSC2.Distance_SP2,8,Port_Data.Data_Transfer[2],0,8)BTD(Q90R2KD.Write.SSC2.Distance_SP2,0,Port_Data.Data_Transfer[3],0,8)BTD(Q90R2KD.Write.SSC2.Distance_Hysteresis,8,Port_Data.Data_Transfer[4],0,8)BTD(Q90R2KD.Write.SSC2.Distance_Hysteresis,0,Port_Data.Data_Transfer[5],0,8)BTD(Q90R2KD.Write.SSC2.Y_SP1,8,Port_Data.Data_Transfer[6],0,8)BTD(Q90R2KD.Write.SSC2.Y_SP1,0,Port_Data.Data_Transfer[7],0,8)BTD(Q90R2KD.Write.SSC2.Y_SP2,8,Port_Data.Data_Transfer[8],0,8)BTD(Q90R2KD.Write.SSC2.Y_SP2,0,Port_Data.Data_Transfer[9],0,8)BTD(Q90R2KD.Write.SSC2.Y_Hysteresis,8,Port_Data.Data_Transfer[10],0,8)BTD(Q90R2KD.Write.SSC2.Y_Hysteresis,0,Port_Data.Data_Transfer[11],0,8)MOV(Port,Port_Data.Data_Transfer[185])MOV(0,Port_Data.Data_Transfer[187])MOV(131,Port_Data.Data_Transfer[188])MOV(12,Port_Data.Data_Transfer[189])MOV(7,Inprocess_Index)OTL(Port_Data.Port_Write.[Port])OTL(Local_Control.11);
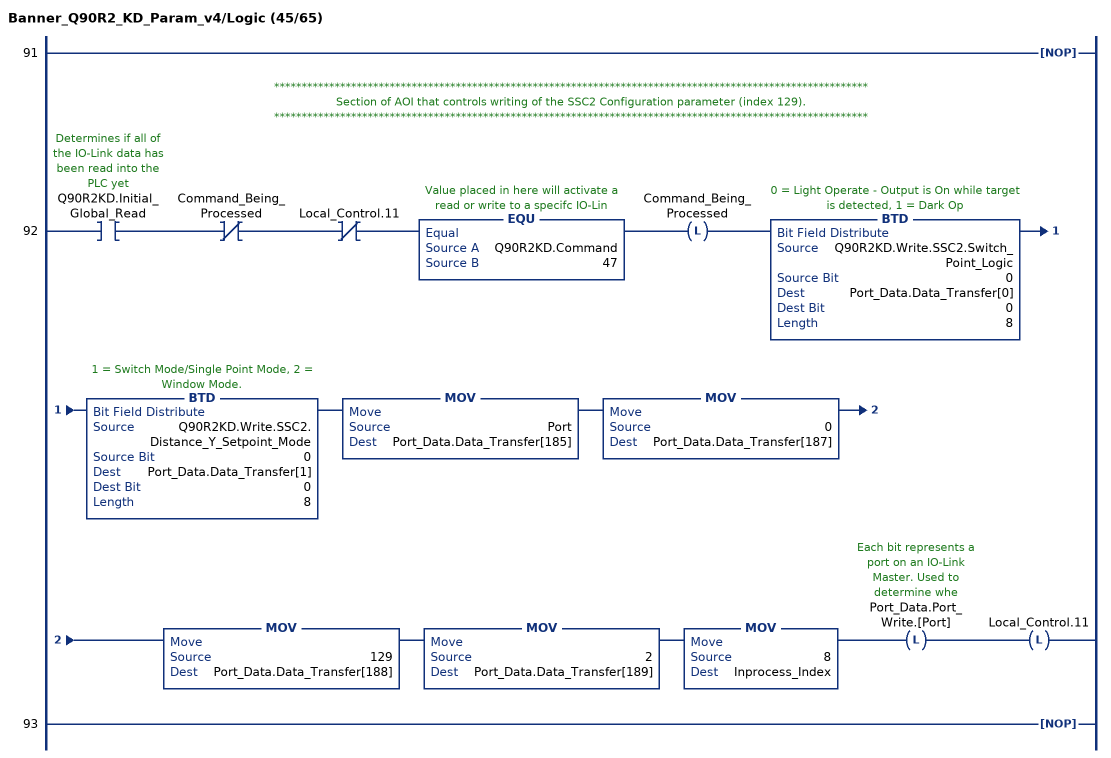
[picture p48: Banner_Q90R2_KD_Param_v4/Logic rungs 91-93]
   91: NOP();
   // ************************************************************************************************************
   // Section of AOI that controls writing of the SSC2 Configuration parameter (index 129).
   // ************************************************************************************************************
   92: XIC(Q90R2KD.Initial_Global_Read)XIO(Command_Being_Processed)XIO(Local_Control.11)EQU(Q90R2KD.Command,47)OTL(Command_Being_Processed)BTD(Q90R2KD.Write.SSC2.Switch_Point_Logic,0,Port_Data.Data_Transfer[0],0,8)BTD(Q90R2KD.Write.SSC2.Distance_Y_Setpoint_Mode,0,Port_Data.Data_Transfer[1],0,8)MOV(Port,Port_Data.Data_Transfer[185])MOV(0,Port_Data.Data_Transfer[187])MOV(129,Port_Data.Data_Transfer[188])MOV(2,Port_Data.Data_Transfer[189])MOV(8,Inprocess_Index)OTL(Port_Data.Port_Write.[Port])OTL(Local_Control.11);
   93: NOP();
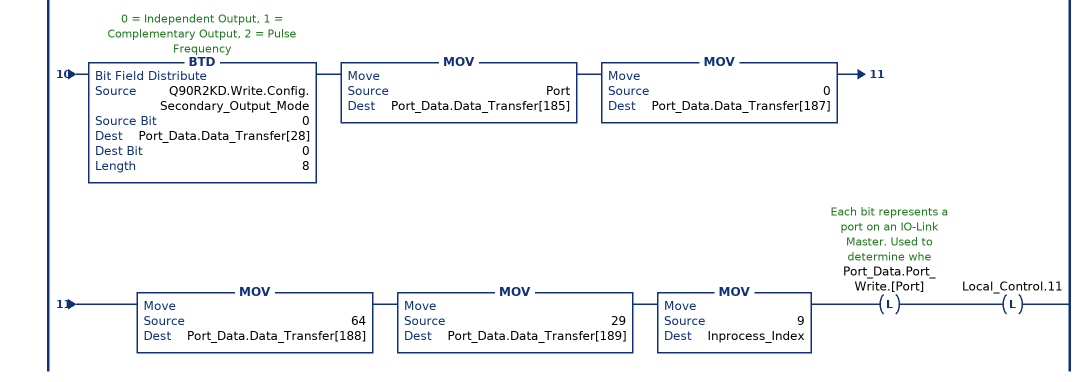
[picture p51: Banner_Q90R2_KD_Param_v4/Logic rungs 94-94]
   // ************************************************************************************************************
   // Section of AOI that controls writing of the Configuration parameter (index 64).
   // ************************************************************************************************************
   94: XIC(Q90R2KD.Initial_Global_Read)XIO(Command_Being_Processed)XIO(Local_Control.11)EQU(Q90R2KD.Command,48)OTL(Command_Being_Processed)BTD(Q90R2KD.Write.Config.Response_Speed,0,Port_Data.Data_Transfer[0],0,8)BTD(Q90R2KD.Write.Config.Detection_Sensitivity,0,Port_Data.Data_Transfer[1],0,8)BTD(Q90R2KD.Write.Config.LEDs_Disabled,0,Port_Data.Data_Transfer[2],0,8)BTD(Q90R2KD.Write.Config.Output_Polarity,0,Port_Data.Data_Transfer[3],0,8)BTD(Q90R2KD.Write.Config.Process_Data_Measurement,0,Port_Data.Data_Transfer[4],0,8)BTD(Q90R2KD.Write.Config.Remote_Input_Mode,0,Port_Data.Data_Transfer[5],0,8)BTD(Q90R2KD.Write.Config.Amplitude_Threshold,24,Port_Data.Data_Transfer[6],0,8)BTD(Q90R2KD.Write.Config.Amplitude_Threshold,16,Port_Data.Data_Transfer[7],0,8)BTD(Q90R2KD.Write.Config.Amplitude_Threshold,8,Port_Data.Data_Transfer[8],0,8)BTD(Q90R2KD.Write.Config.Amplitude_Threshold,0,Port_Data.Data_Transfer[9],0,8)BTD(Q90R2KD.Write.Config.Limit_Filter_Enabled,0,Port_Data.Data_Transfer[10],0,8)BTD(Q90R2KD.Write.Config.Limit_Filter_Positive_Hold_Time,24,Port_Data.Data_Transfer[11],0,8)BTD(Q90R2KD.Write.Config.Limit_Filter_Positive_Hold_Time,16,Port_Data.Data_Transfer[12],0,8)BTD(Q90R2KD.Write.Config.Limit_Filter_Positive_Hold_Time,8,Port_Data.Data_Transfer[13],0,8)BTD(Q90R2KD.Write.Config.Limit_Filter_Positive_Hold_Time,0,Port_Data.Data_Transfer[14],0,8)BTD(Q90R2KD.Write.Config.Limit_Filter_Negative_Hold_Time,24,Port_Data.Data_Transfer[15],0,8)BTD(Q90R2KD.Write.Config.Limit_Filter_Negative_Hold_Time,16,Port_Data.Data_Transfer[16],0,8)BTD(Q90R2KD.Write.Config.Limit_Filter_Negative_Hold_Time,8,Port_Data.Data_Transfer[17],0,8)BTD(Q90R2KD.Write.Config.Limit_Filter_Negative_Hold_Time,0,Port_Data.Data_Transfer[18],0,8)BTD(Q90R2KD.Write.Config.Limit_Filter_Positive_Distance,24,Port_Data.Data_Transfer[19],0,8)BTD(Q90R2KD.Write.Config.Limit_Filter_Positive_Distance,16,Port_Data.Data_Transfer[20],0,8)BTD(Q90R2KD.Write.Config.Limit_Filter_Positive_Distance,8,Port_Data.Data_Transfer[21],0,8)BTD(Q90R2KD.Write.Config.Limit_Filter_Positive_Distance,0,Port_Data.Data_Transfer[22],0,8)BTD(Q90R2KD.Write.Config.Limit_Filter_Negative_Distance,24,Port_Data.Data_Transfer[23],0,8)BTD(Q90R2KD.Write.Config.Limit_Filter_Negative_Distance,16,Port_Data.Data_Transfer[24],0,8)BTD(Q90R2KD.Write.Config.Limit_Filter_Negative_Distance,8,Port_Data.Data_Transfer[25],0,8)BTD(Q90R2KD.Write.Config.Limit_Filter_Negative_Distance,0,Port_Data.Data_Transfer[26],0,8)BTD(Q90R2KD.Write.Config.Primary_Output_Mode,0,Port_Data.Data_Transfer[27],0,8)BTD(Q90R2KD.Write.Config.Secondary_Output_Mode,0,Port_Data.Data_Transfer[28],0,8)MOV(Port,Port_Data.Data_Transfer[185])MOV(0,Port_Data.Data_Transfer[187])MOV(64,Port_Data.Data_Transfer[188])MOV(29,Port_Data.Data_Transfer[189])MOV(9,Inprocess_Index)OTL(Port_Data.Port_Write.[Port])OTL(Local_Control.11);
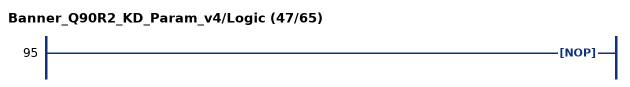
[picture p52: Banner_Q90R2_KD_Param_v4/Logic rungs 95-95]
   95: NOP();
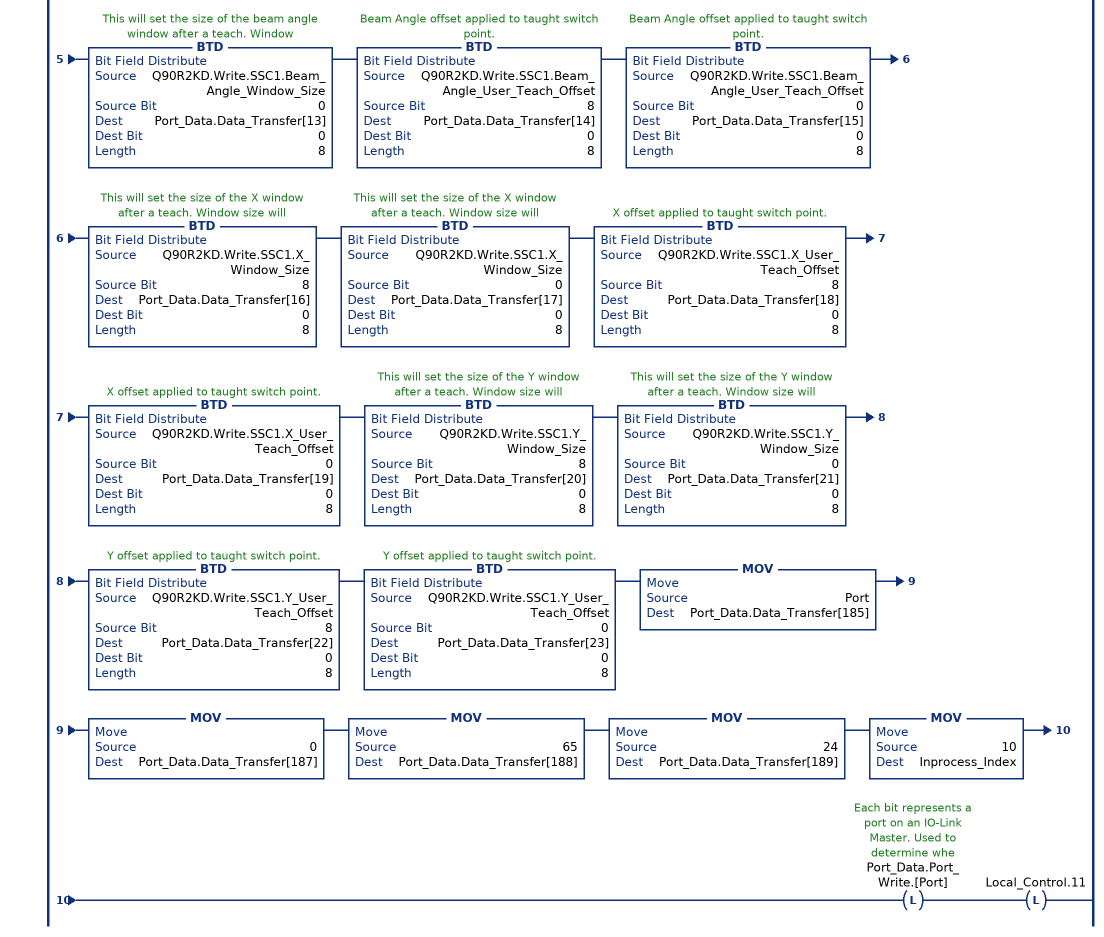
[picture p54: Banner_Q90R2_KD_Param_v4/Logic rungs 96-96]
   // ************************************************************************************************************
   // Section of AOI that controls writing of the SSC1 Vendor Specific Configuration parameter (index 65).
   // ************************************************************************************************************
   96: XIC(Q90R2KD.Initial_Global_Read)XIO(Command_Being_Processed)XIO(Local_Control.11)EQU(Q90R2KD.Command,49)OTL(Command_Being_Processed)BTD(Q90R2KD.Write.SSC1.Delay_On,24,Port_Data.Data_Transfer[0],0,8)BTD(Q90R2KD.Write.SSC1.Delay_On,16,Port_Data.Data_Transfer[1],0,8)BTD(Q90R2KD.Write.SSC1.Delay_On,8,Port_Data.Data_Transfer[2],0,8)BTD(Q90R2KD.Write.SSC1.Delay_On,0,Port_Data.Data_Transfer[3],0,8)BTD(Q90R2KD.Write.SSC1.Delay_Off,24,Port_Data.Data_Transfer[4],0,8)BTD(Q90R2KD.Write.SSC1.Delay_Off,16,Port_Data.Data_Transfer[5],0,8)BTD(Q90R2KD.Write.SSC1.Delay_Off,8,Port_Data.Data_Transfer[6],0,8)BTD(Q90R2KD.Write.SSC1.Delay_Off,0,Port_Data.Data_Transfer[7],0,8)BTD(Q90R2KD.Write.SSC1.Distance_Window_Size,8,Port_Data.Data_Transfer[8],0,8)BTD(Q90R2KD.Write.SSC1.Distance_Window_Size,0,Port_Data.Data_Transfer[9],0,8)BTD(Q90R2KD.Write.SSC1.Distance_User_Teach_Offset,8,Port_Data.Data_Transfer[10],0,8)BTD(Q90R2KD.Write.SSC1.Distance_User_Teach_Offset,0,Port_Data.Data_Transfer[11],0,8)BTD(Q90R2KD.Write.SSC1.Beam_Angle_Window_Size,8,Port_Data.Data_Transfer[12],0,8)BTD(Q90R2KD.Write.SSC1.Beam_Angle_Window_Size,0,Port_Data.Data_Transfer[13],0,8)BTD(Q90R2KD.Write.SSC1.Beam_Angle_User_Teach_Offset,8,Port_Data.Data_Transfer[14],0,8)BTD(Q90R2KD.Write.SSC1.Beam_Angle_User_Teach_Offset,0,Port_Data.Data_Transfer[15],0,8)BTD(Q90R2KD.Write.SSC1.X_Window_Size,8,Port_Data.Data_Transfer[16],0,8)BTD(Q90R2KD.Write.SSC1.X_Window_Size,0,Port_Data.Data_Transfer[17],0,8)BTD(Q90R2KD.Write.SSC1.X_User_Teach_Offset,8,Port_Data.Data_Transfer[18],0,8)BTD(Q90R2KD.Write.SSC1.X_User_Teach_Offset,0,Port_Data.Data_Transfer[19],0,8)BTD(Q90R2KD.Write.SSC1.Y_Window_Size,8,Port_Data.Data_Transfer[20],0,8)BTD(Q90R2KD.Write.SSC1.Y_Window_Size,0,Port_Data.Data_Transfer[21],0,8)BTD(Q90R2KD.Write.SSC1.Y_User_Teach_Offset,8,Port_Data.Data_Transfer[22],0,8)BTD(Q90R2KD.Write.SSC1.Y_User_Teach_Offset,0,Port_Data.Data_Transfer[23],0,8)MOV(Port,Port_Data.Data_Transfer[185])MOV(0,Port_Data.Data_Transfer[187])MOV(65,Port_Data.Data_Transfer[188])MOV(24,Port_Data.Data_Transfer[189])MOV(10,Inprocess_Index)OTL(Port_Data.Port_Write.[Port])OTL(Local_Control.11);
